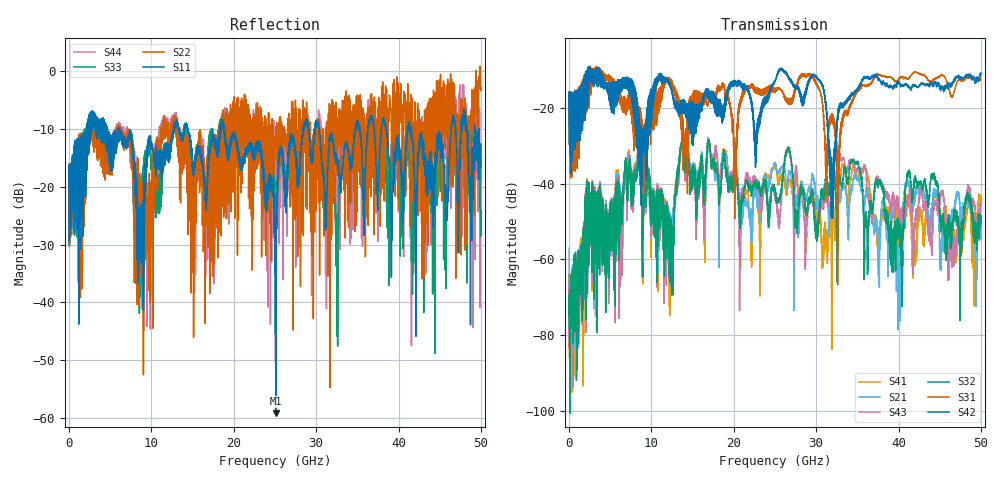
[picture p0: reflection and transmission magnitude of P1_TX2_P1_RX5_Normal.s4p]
!Keysight Technologies,N5225B,MY57041031,A.13.20.10
!Date: Friday, May 31, 2019 11:20:36
!Correction: S11(Full 4 Port(1,2,3,4))
!S12(Full 4 Port(1,2,3,4))
!S13(Full 4 Port(1,2,3,4))
!S14(Full 4 Port(1,2,3,4))
!S21(Full 4 Port(1,2,3,4))
!S22(Full 4 Port(1,2,3,4))
!S23(Full 4 Port(1,2,3,4))
!S24(Full 4 Port(1,2,3,4))
!S31(Full 4 Port(1,2,3,4))
!S32(Full 4 Port(1,2,3,4))
!S33(Full 4 Port(1,2,3,4))
!S34(Full 4 Port(1,2,3,4))
!S41(Full 4 Port(1,2,3,4))
!S42(Full 4 Port(1,2,3,4))
!S43(Full 4 Port(1,2,3,4))
!S44(Full 4 Port(1,2,3,4))
!S4P File: Measurements: <S11,S12,S13,S14>,
!<S21,S22,S23,S24>,
!<S31,S32,S33,S34>,
!<S41,S42,S43,S44>:
# Hz S  dB  R 50.0
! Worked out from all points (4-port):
!   5000 points, 10 MHz to 50 GHz, reference 50 ohm
!   strongest paths, dB at 10 MHz, 12.51 GHz, 25.01 GHz, 37.51 GHz, 50 GHz:
!     S42: -19.4, -15.7, -13.0, -12.4, -10.9
!     S31: -19.4, -13.0, -15.4, -11.2, -12.5
!     S32: -78.2, -53.1, -41.6, -40.4, -48.5
!     S43: -72.3, -56.2, -43.2, -38.6, -44.9
!     S21: -57.0, -49.2, -34.3, -54.4, -54.6
!     S41: -72.7, -51.1, -35.3, -56.6, -44.6
!   lowest |S11| = -59.2 dB at 25.1 GHz (marker M1), VSWR 1.00, Z = 49.9 - j0.0401 ohm
!   |S11| at or under -10 dB: 6.091 GHz to 12.71 GHz (6.616 GHz wide, 70.4 % of centre); 18.82 GHz to 28.43 GHz (9.605 GHz wide, 40.7 % of centre); 41.58 GHz to 46.39 GHz (4.81 GHz wide, 10.9 % of centre)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
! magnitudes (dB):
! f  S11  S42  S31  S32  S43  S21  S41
! 10 MHz  -19.8  -19.4  -19.4  -78.2  -72.3  -57.0  -72.7
! 8.41 GHz  -24.7  -21.6  -24.6  -33.5  -33.6  -32.1  -32.1
! 12.28 GHz  -14.0  -13.7  -12.6  -61.6  -57.3  -61.6  -63.0
! 13.66 GHz  -11.1  -20.4  -21.7  -29.1  -29.3  -29.1  -29.2
! 25.1 GHz  -59.2  -12.3  -15.1  -42.5  -42.6  -35.2  -35.2
! 31.94 GHz  -11.0  -36.3  -22.1  -38.9  -36.0  -43.8  -56.6
! 50 GHz  -12.7  -10.9  -12.5  -48.5  -44.9  -54.6  -44.6
